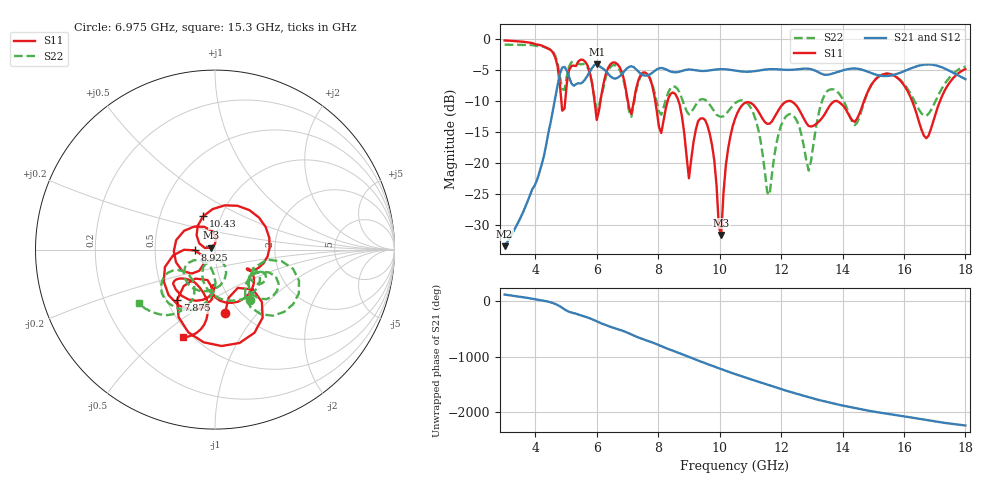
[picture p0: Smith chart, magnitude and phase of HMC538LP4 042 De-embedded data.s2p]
! Chelmsford, MA 01824
! http://www.hittite.com
! Tel: 978-250-3343
! Fax: 978-250-3373
! Device  :  HMC538LP4
! Description:  600 Analog Phase Shifter
! Frequency  :  6.0 GHz - 15.0 GHz
! Package  :  LP4  - 4x4 mm Quad Flatpack No-Lead (QFN) Plastic Package: 24 pin
! Ports  :  2 RF, 1 DC
!  Pin  3  = Rfin  = Port 1
!  Pin  16  = Rfout = Port 2
!  pin  21  = vCTL
! Voltages:  VCTL  = 0 to 5.0 Volts
! Currents :  Vb(V)  Vd(V)  Ib(mA)  Id(mA)
!  0.00  4.20  0.000000	0.479981
! Data:  The device was measured on evaluation board 111296-1.
!  Data was collected using a calibrated network analyzer.
!  The evaluation circuit board was modeled and simulated.This was use
!  to removed the evaluation board circuit from the measured data.
!  The reference plane is the center of the package pin.
! Misc:  Lot #
!Date Measured:  03 - 11 -2009
! Date:  03 - 17 -2009
! Note:
!  Hittite Microwave supplies this data as a sample of measured data at the
!  package pin for this package product.  Your particular data for this product
!  may vary.
!  Data was taken at 25 degrees C.
!  Hittite Microwave reserves the right to change this data at anytime.
# MHz S MA R 50
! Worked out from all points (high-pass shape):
!   201 points, 3 GHz to 18 GHz, reference 50 ohm
!   highest |S21| = -4.03 dB at 6 GHz (marker M1); lowest = -33.5 dB at 3 GHz (marker M2)
!   |S21| within 3 dB of the highest: 4.742 GHz to 5.166 GHz (424.4 MHz wide, 8.57 % of centre); 5.517 GHz to end of sweep
!   lowest |S11| = -31.7 dB at 10.05 GHz (marker M3), VSWR 1.05, Z = 47.7 + j1.03 ohm
!   |S11| at or under -10 dB: 8.66 GHz to 12.22 GHz (3.56 GHz wide, 34.1 % of centre); 12.31 GHz to 13.77 GHz (1.456 GHz wide, 11.2 % of centre); 16.27 GHz to 17.17 GHz (906.1 MHz wide, 5.42 % of centre)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
!   |S22| runs from -25.2 to -0.9 dB; largest |S21 - S12| = 0.0027
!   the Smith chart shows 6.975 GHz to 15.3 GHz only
!   S11 on the Smith chart (normalised r, x): 6.975 GHz: 0.86, -0.70; 7.875 GHz: 0.57, -0.36; 8.925 GHz: 0.80, -0.01; 10.43 GHz: 0.82, +0.32; 15.3 GHz: 0.45, -0.60
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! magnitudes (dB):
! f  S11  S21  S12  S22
! 3 GHz  -0.2  -33.5  -33.5  -0.9
! 4.575 GHz  -2.2  -11.5  -11.5  -2.0
! 4.875 GHz  -11.6  -4.6  -4.6  -8.1
! 5.55 GHz  -3.3  -6.9  -6.9  -4.0
! 6 GHz  -13.0  -4.0  -4.0  -11.4
! 6.45 GHz  -4.0  -6.0  -6.0  -4.4
! 6.975 GHz  -8.9  -4.7  -4.7  -9.3
! 7.875 GHz  -9.1  -5.2  -5.2  -8.5
! 8.025 GHz  -14.2  -4.7  -4.7  -11.7
! 8.55 GHz  -8.8  -5.3  -5.4  -7.7
! 8.925 GHz  -19.0  -4.9  -4.9  -11.6
! 9.525 GHz  -13.0  -5.1  -5.1  -9.8
! 10.05 GHz  -31.7  -4.8  -4.8  -12.5
! 10.43 GHz  -14.1  -5.0  -5.0  -10.7
! 10.5 GHz  -12.9  -5.1  -5.1  -10.3
! 11.62 GHz  -13.7  -4.8  -4.8  -25.2
! 12.15 GHz  -10.1  -4.9  -5.0  -12.5
! 13.05 GHz  -14.0  -5.0  -5.0  -17.1
! 15.3 GHz  -5.7  -5.9  -6.0  -5.7
! 15.53 GHz  -5.6  -5.9  -5.9  -5.6
! 16.73 GHz  -16.0  -4.1  -4.1  -12.4
! 18 GHz  -4.8  -6.5  -6.5  -4.4
